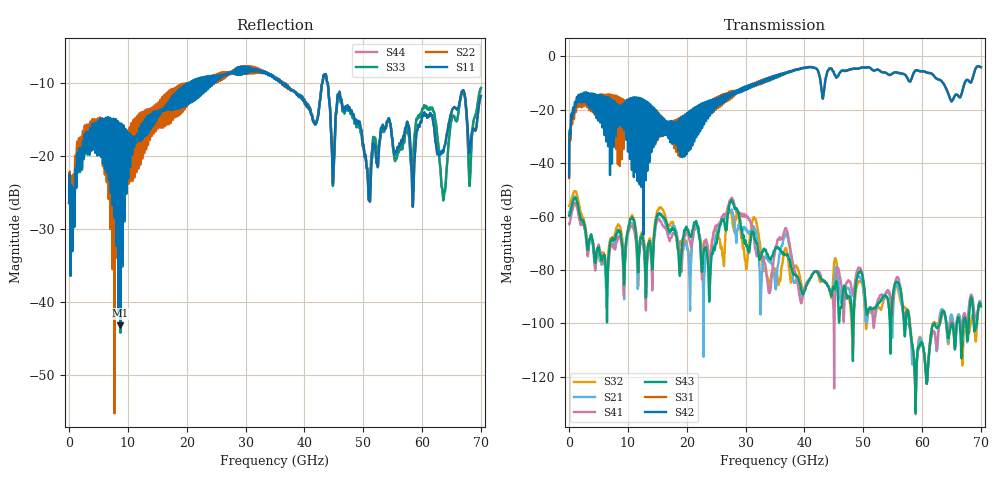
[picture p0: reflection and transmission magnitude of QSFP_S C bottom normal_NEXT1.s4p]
! AWR Design Environment (8415) Tue Jan 08 12:44:44 2019
! Document = 'QSFP Channel_S'
! nPorts: 4, nXvals: 7001
# HZ S DB R 50
!Freq DBS11 AngS11 DBS12 AngS12 DBS13 AngS13 DBS14 AngS14
!	DBS21 AngS21 DBS22 AngS22 DBS23 AngS23 DBS24 AngS24
!	DBS31 AngS31 DBS32 AngS32 DBS33 AngS33 DBS34 AngS34
!	DBS41 AngS41 DBS42 AngS42 DBS43 AngS43 DBS44 AngS44
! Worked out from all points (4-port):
!   7000 points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, 10 MHz to 70 GHz, reference 50 ohm
!   strongest paths, dB at 10 MHz, 17.51 GHz, 35.01 GHz, 52.51 GHz, 70 GHz:
!     S42: -45.0, -30.3, -7.3, -5.0, -4.0
!     S31: -45.6, -27.8, -7.4, -5.0, -4.0
!     S43: -59.7, -64.7, -72.2, -92.5, -93.6
!     S41: -62.9, -67.1, -73.4, -91.0, -93.2
!     S21: -58.5, -64.0, -85.1, -92.5, -92.6
!     S32: -56.0, -62.1, -79.7, -93.8, -93.1
!   lowest |S11| = -43.2 dB at 8.73 GHz (marker M1), VSWR 1.01, Z = 49.5 - j0.488 ohm
!   |S11| at or under -10 dB: start of sweep to 20.43 GHz; 36.44 GHz to 43.04 GHz (6.602 GHz wide, 16.6 % of centre); 43.96 GHz to end of sweep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
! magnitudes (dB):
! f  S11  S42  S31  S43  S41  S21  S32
! 10 MHz  -26.4  -45.0  -45.6  -59.7  -62.9  -58.5  -56.0
! 1.63 GHz  -20.1  -14.4  -15.6  -57.6  -60.0  -57.4  -54.8
! 8.73 GHz  -43.2  -21.1  -17.0  -66.0  -67.9  -66.4  -64.2
! 23.86 GHz  -9.8  -18.4  -17.8  -91.1  -81.0  -73.1  -79.2
! 27.63 GHz  -8.5  -14.8  -15.7  -53.8  -52.9  -57.4  -59.3
! 33.8 GHz  -8.9  -9.2  -9.2  -74.4  -86.2  -75.8  -83.5
! 70 GHz  -11.8  -4.0  -4.0  -93.6  -93.2  -92.6  -93.1
